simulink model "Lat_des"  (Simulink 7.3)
settings: Solver=ode45  StartTime=0.0  StopTime=10.0  RelTol=1e-3
undefined symbols (not defined in the file or in its folder): Al, Bl, Cl, Dl

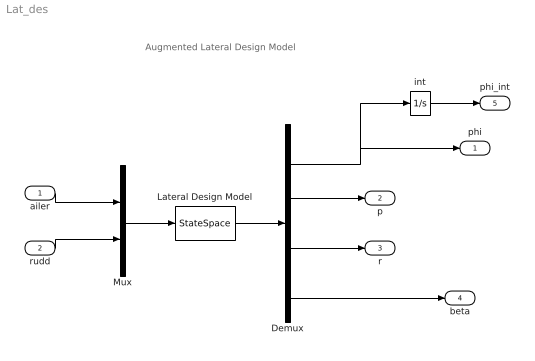
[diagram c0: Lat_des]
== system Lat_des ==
  note: Augmented Lateral Design Model
  ailer : Inport  OutDataType=sfix(16)  OutScaling=2^0
  rudd : Inport  Port=2  OutDataType=sfix(16)  OutScaling=2^0
  Demux : Demux
  Lateral Design Model : StateSpace  A=Al  B=Bl  C=Cl  D=Dl
  Mux : Mux  Inputs=2
  int : Integrator
  phi : Outport  OutDataType=sfix(16)  OutScaling=2^0
  p : Outport  Port=2  OutDataType=sfix(16)  OutScaling=2^0
  r : Outport  Port=3  OutDataType=sfix(16)  OutScaling=2^0
  beta : Outport  Port=4  OutDataType=sfix(16)  OutScaling=2^0
  phi_int : Outport  Port=5  OutDataType=sfix(16)  OutScaling=2^0
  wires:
  Mux/1 -> Lateral Design Model/1
  ailer/1 -> Mux/1
  rudd/1 -> Mux/2
  Demux/1 -> phi/1, int/1
  Demux/2 -> p/1
  int/1 -> phi_int/1
  Demux/3 -> r/1
  Demux/4 -> beta/1
  Lateral Design Model/1 -> Demux/1
